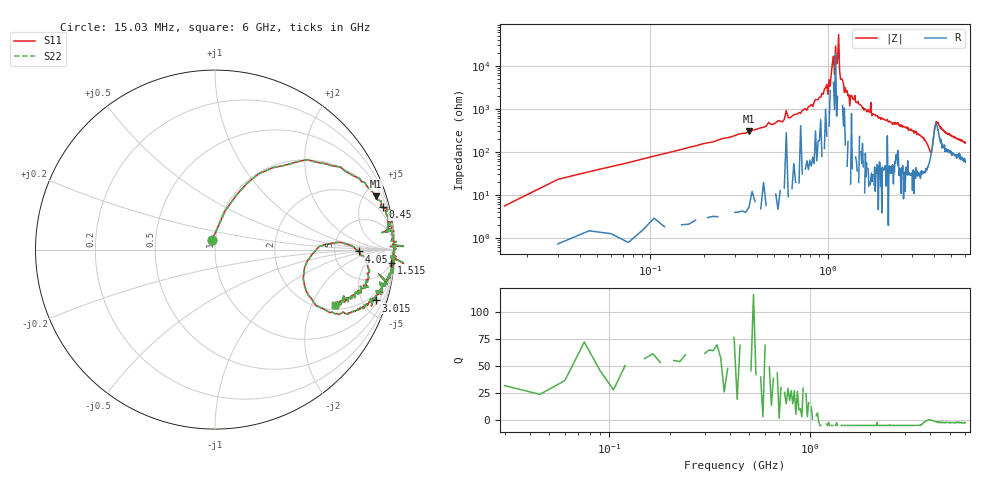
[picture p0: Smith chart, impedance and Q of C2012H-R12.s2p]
!	Network	Analyzer	HP8753E.07.74:	Oct	30	2002	Serial	No.	JP38451487
!	Hewlett-Packard
!	28	Aug	2009	10:41:15
!	Frequency	S11	S21	S12	S22
#	HZ	S	RI	R	50
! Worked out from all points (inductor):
!   400 points, 15.03 MHz to 6 GHz, reference 50 ohm
!   read as one part in series: L = 120 nH near 45.03 MHz
!   highest Q = 61.4 at 360 MHz (marker M1), where L = 132 nH
!   self-resonance near 1.095 GHz
!   S11 on the Smith chart (normalised r, x): 15.03 MHz: 0.96, +0.10; 450 MHz: 1.11, +7.91; 1.515 GHz: 6, -25; 3.015 GHz: 1.25, -6.25; 4.05 GHz: 9.17, -0.55; 6 GHz: 2.22, -3.03
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1.502992e7  -0.0161 0.0536  1.02 -0.0536  1.02 -0.0536  -0.0161 0.0536
3.002985e7  0.0563 0.215  0.944 -0.215  0.944 -0.215  0.0563 0.215
9.002955e7  0.321 0.456  0.679 -0.456  0.679 -0.456  0.321 0.456
3.600282e8  0.895 0.298  0.105 -0.298  0.105 -0.298  0.895 0.298
4.500278e8  0.937 0.236  0.0631 -0.236  0.0631 -0.236  0.937 0.236
1.005025e9  1.05 0.0179  -0.045 -0.0179  -0.045 -0.0179  1.05 0.0179
1.020025e9  0.998 0.0206  0.00214 -0.0206  0.00214 -0.0206  0.998 0.0206
1.080025e9  0.999 0.00577  0.0015 -0.00577  0.0015 -0.00577  0.999 0.00577
1.095025e9  0.997 0.0156  0.00262 -0.0156  0.00262 -0.0156  0.997 0.0156
1.110024e9  0.998 -0.0025  0.00238 0.0025  0.00238 0.0025  0.998 -0.0025
1.140024e9  0.999 -0.00702  0.00104 0.00702  0.00104 0.00702  0.999 -0.00702
1.155024e9  1 -0.0014  -0.00122 0.0014  -0.00122 0.0014  1 -0.0014
1.170024e9  1 -0.013  0 0.013  0 0.013  1 -0.013
1.245024e9  0.981 -0.036  0.0192 0.036  0.0192 0.036  0.981 -0.036
1.515022e9  0.98 -0.0751  0.0198 0.0751  0.0198 0.0751  0.98 -0.0751
2.01002e9  0.964 -0.155  0.0356 0.155  0.0356 0.155  0.964 -0.155
3.015015e9  0.898 -0.283  0.102 0.283  0.102 0.283  0.898 -0.283
3.795011e9  0.508 -0.229  0.492 0.229  0.492 0.229  0.508 -0.229
4.00501e9  0.759 0.0218  0.241 -0.0218  0.241 -0.0218  0.759 0.0218
4.05001e9  0.804 -0.0105  0.196 0.0105  0.196 0.0105  0.804 -0.0105
5.010005e9  0.778 -0.256  0.222 0.256  0.222 0.256  0.778 -0.256
6e9  0.671 -0.31  0.329 0.31  0.329 0.31  0.671 -0.31
